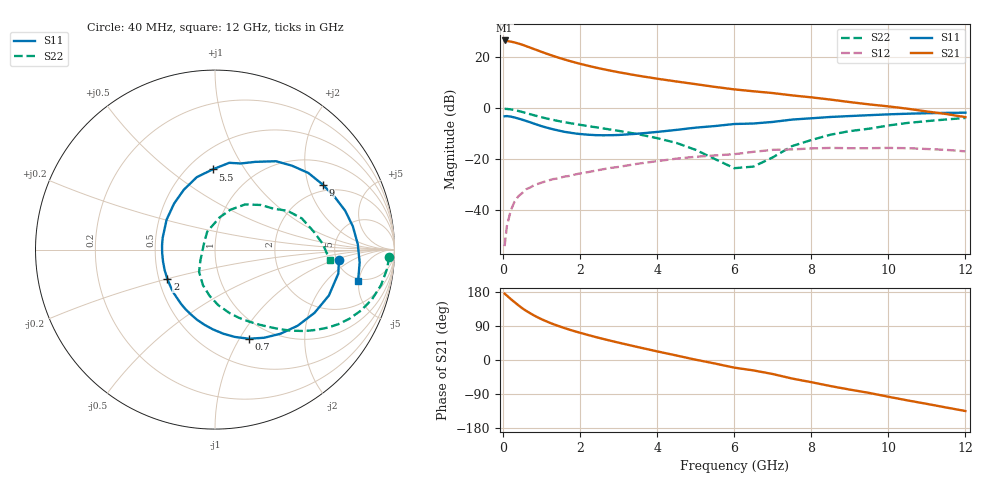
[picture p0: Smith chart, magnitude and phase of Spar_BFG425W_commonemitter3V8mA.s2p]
! Filename: 38bfg425.001
! BFG425W Field C1
! V1=8.355E-001V,V2=3.000E+000V, I1=1.001E-004A, I2=8.000E-003A
# GHz  S  MA  R 50
!  S11  S21  S12  S22
!Freq(GHz)  Mag  Ang  Mag  Ang  Mag  Ang  Mag  Ang
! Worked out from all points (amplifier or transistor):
!   44 points, 40 MHz to 12 GHz, reference 50 ohm
!   highest |S21| = 26.5 dB at 40 MHz (marker M1)
!   |S21| within 3 dB of that: start of sweep to 738.7 MHz
!   unconditionally stable (mu >= 1): 2.08 GHz to end of sweep
!   at 700 MHz: K = 0.46, MSG = 27.4 dB, |S12| = -31.1 dB
!   at 2.4 GHz: K = 1.07, MAG = 18.5 dB, |S12| = -24.4 dB
!   at 12 GHz: K = 1.42, MAG = 2.9 dB, |S12| = -16.9 dB
!   S11 on the Smith chart (normalised r, x): 40 MHz: 5.26, -1.14; 700 MHz: 0.79, -1.10; 2 GHz: 0.55, -0.20; 5.5 GHz: 0.65, +0.73; 9 GHz: 1.75, +2.49; 12 GHz: 4.73, -4.88
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0.04  0.693 -4.6  21.1 175.1  0.002 69.5  0.97 -2.3
0.2  0.684 -22.0  20.05 160.8  0.01 76.5  0.946 -12.1
0.3  0.657 -32.4  19.27 152.4  0.015 72.3  0.917 -17.7
0.4  0.626 -42.7  18.36 144.3  0.019 67.4  0.881 -22.7
0.5  0.594 -52.1  17.4 136.4  0.022 63.4  0.842 -27.2
0.6  0.562 -61.0  16.32 129.7  0.026 59.9  0.803 -31.2
0.7  0.531 -69.2  15.31 123.6  0.028 56.9  0.764 -34.7
0.9  0.471 -84.3  13.46 112.5  0.033 52.5  0.695 -40.5
1.2  0.404 -104.2  11.15 98.8  0.039 48.0  0.612 -47.4
1.4  0.371 -116.1  9.939 91.1  0.042 45.8  0.568 -51.1
1.6  0.344 -127.5  8.931 84.1  0.046 44.1  0.531 -54.5
2  0.312 -148.1  7.372 71.7  0.053 41.1  0.472 -61.0
2.2  0.303 -157.9  6.764 66.2  0.056 39.6  0.447 -64.2
3  0.299 167.0  5.043 45.7  0.071 33.0  0.36 -77.5
3.5  0.317 148.3  4.326 34.1  0.082 27.8  0.31 -86.6
4.5  0.376 117.6  3.324 11.9  0.103 15.3  0.209 -108.8
5.5  0.447 91.7  2.607 -9.4  0.119 1.1  0.101 -143.7
6.5  0.501 73.3  2.138 -27.5  0.14 -9.6  0.072 146.5
8.5  0.673 39.4  1.472 -68.8  0.167 -46.0  0.303 56.2
9  0.701 31.1  1.315 -78.1  0.165 -54.3  0.356 44.3
10.5  0.779 9.5  0.975 -106.7  0.165 -81.4  0.514 19.7
12  0.816 -12.2  0.668 -134.6  0.143 -112.0  0.643 -5.4
